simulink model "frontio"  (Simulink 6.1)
settings: Solver=ode45  StartTime=0.0  StopTime=25.0  RelTol=1e-3
undefined symbols (not defined in the file or in its folder): Bit, frontio_netlist, Location, Lower, Width
libraries: xbsIndex_r3 x12, adlibrary2 x1

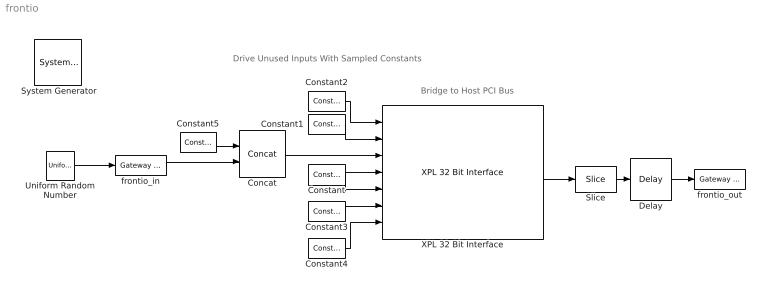
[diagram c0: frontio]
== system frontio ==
  note: Drive Unused Inputs With Sampled Constants
  note: Bridge to Host PCI Bus
  " System Generator" : xbsIndex_r3/ System Generator  Tag=genX  xilinxfamily=Virtex2P  part=xc2vp70  speed=-5  package=ff1704  synthesis_tool=XST  directory=./frontio_netlist  testbench=off  simulink_period=1  sysclk_period=7.5  incr_netlist=off  trim_vbits=Everywhere in SubSystem  dbl_ovrd=According to Block Masks  core_generation=According to Block Masks  run_coregen=off  deprecated_control=off  eval_field=0
  Concat : xbsIndex_r3/Concat  num_inputs=2  explicit_period=off  period=1  dbl_ovrd=off
  Constant : xbsIndex_r3/Constant  const=0  equ=P=C  arith_type=Boolean  n_bits=1  bin_pt=0  opselect=C  inp2=PCIN>>17  opr=+  inp1=P  carry=CIN  iostate=0  explicit_period=on  period=1  dbl_ovrd=off
  Constant1 : xbsIndex_r3/Constant  const=1  equ=P=C  arith_type=Boolean  n_bits=1  bin_pt=0  opselect=C  inp2=PCIN>>17  opr=+  inp1=P  carry=CIN  iostate=0  explicit_period=on  period=1  dbl_ovrd=off
  Constant2 : xbsIndex_r3/Constant  const=0  equ=P=C  arith_type=Unsigned  n_bits=32  bin_pt=0  opselect=C  inp2=PCIN>>17  opr=+  inp1=P  carry=CIN  iostate=0  explicit_period=on  period=1  dbl_ovrd=off
  Constant3 : xbsIndex_r3/Constant  const=0  equ=P=C  arith_type=Unsigned  n_bits=32  bin_pt=0  opselect=C  inp2=PCIN>>17  opr=+  inp1=P  carry=CIN  iostate=0  explicit_period=on  period=1  dbl_ovrd=off
  Constant4 : xbsIndex_r3/Constant  const=0  equ=P=C  arith_type=Unsigned  n_bits=66  bin_pt=0  opselect=C  inp2=PCIN>>17  opr=+  inp1=P  carry=CIN  iostate=0  explicit_period=on  period=1  dbl_ovrd=off
  Constant5 : xbsIndex_r3/Constant  const=0  equ=P=C  arith_type=Unsigned  n_bits=24  bin_pt=0  opselect=C  inp2=PCIN>>17  opr=+  inp1=P  carry=CIN  iostate=0  explicit_period=on  period=1  dbl_ovrd=off
  Delay : xbsIndex_r3/Delay  latency=1  reg_retiming=off  explicit_period=on  period=1  en=off  accept_only_valid=off  init_zero=on  dbl_ovrd=off  show_param=off
  Slice : xbsIndex_r3/Slice  mode=Lower Bit Location + Width  nbits=8  bit1=0  base1=MSB of Input  bit0=0  base0=LSB of Input  boolean_output=off  explicit_period=off  period=1  dbl_ovrd=off
  Uniform Random Number : UniformRandomNumber  SampleTime=0
  XPL 32 Bit Interface : adlibrary2/ADM-XPL/XPL 32 Bit Interface  program=''  clock_ratio=1.5
  frontio_in : xbsIndex_r3/Gateway In  arith_type=Unsigned  n_bits=8  bin_pt=0  quantization=Truncate  overflow=Wrap  period=1  timing_constraint=None  locs_specified=on  LOCs={'D10','C13','E10','D13','F11','H13','E11','G13'}  needs_fixed_name=off  dbl_ovrd=off  show_param=off
  frontio_out : xbsIndex_r3/Gateway Out  output_type=Double  nbits=8  bin_pt=6  arith_type=Boolean  quantization=Truncate  overflow=Wrap  hdl_port=on  timing_constraint=None  locs_specified=on  LOCs={'J10','M19','H10','L19','G10','L18','F10','K18'}  needs_fixed_name=off  show_param=off
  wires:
  Constant/1 -> XPL 32 Bit Interface/4, XPL 32 Bit Interface/5
  Constant1/1 -> XPL 32 Bit Interface/2
  Constant2/1 -> XPL 32 Bit Interface/1
  Constant3/1 -> XPL 32 Bit Interface/6
  Constant4/1 -> XPL 32 Bit Interface/7
  XPL 32 Bit Interface/6 -> Slice/1
  Delay/1 -> frontio_out/1
  Slice/1 -> Delay/1
  frontio_in/1 -> Concat/2
  Concat/1 -> XPL 32 Bit Interface/3
  Constant5/1 -> Concat/1
  Uniform Random Number/1 -> frontio_in/1
